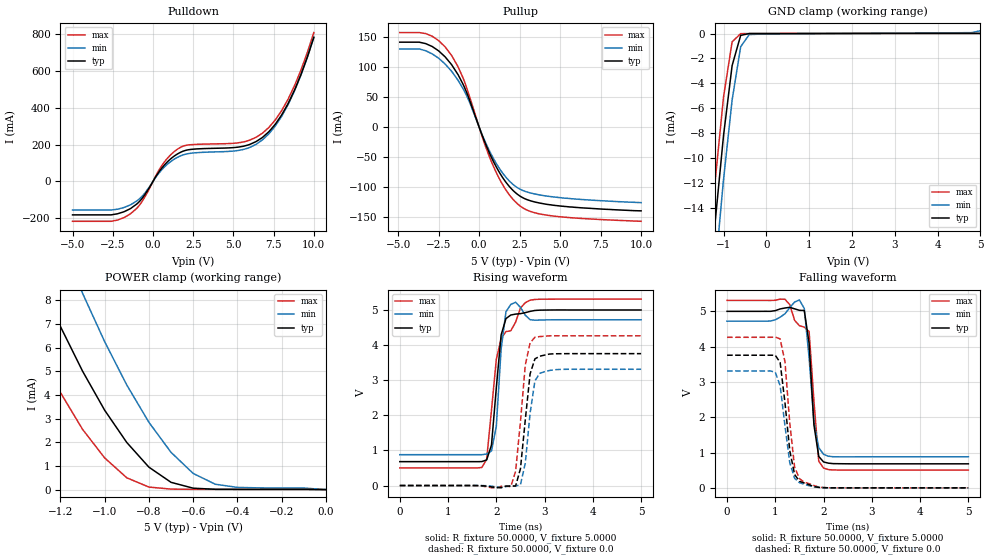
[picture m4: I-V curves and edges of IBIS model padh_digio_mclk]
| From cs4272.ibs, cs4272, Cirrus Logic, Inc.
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|   Model mclk
[Model]  padh_digio_mclk
Model_type I/O
Polarity   Non-Inverting
Enable   Active-High
Vinl =   0.8000V
Vinh =   2.0000V
C_comp   5.0000pF   5.0000pF   5.0000pF
[Temperature Range]   25.0000   85.0000   -40.0000
[Voltage Range]   5.0000V   4.5000V   5.5000V
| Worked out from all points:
|   slope of the pulldown table from 0 to 0.75 V, typ, clamps not added: 8.05 ohm
|   slope of the pullup table from 0 to 0.75 V, typ, clamps not added: 15.1 ohm
|   GND clamp passes 1 mA (typ) near -0.67 V on its own axis
|   POWER clamp passes 1 mA (typ) near -0.81 V on its own axis
|   rising waveform, R_fixture 50.0000, V_fixture 5.0000: 20-80 % time 166ps typ, 112ps min, 330ps max; typ from 0.681 V to 5 V
|   rising waveform, R_fixture 50.0000, V_fixture 0.0: 20-80 % time 167ps typ, 162ps min, 167ps max; typ from 0 V to 3.76 V
|   falling waveform, R_fixture 50.0000, V_fixture 5.0000: 20-80 % time 131ps typ, 149ps min, 154ps max; typ from 5 V to 0.681 V
|   falling waveform, R_fixture 50.0000, V_fixture 0.0: 20-80 % time 197ps typ, 189ps min, 169ps max; typ from 3.76 V to 0 V
[Pulldown]
|Voltage   I(typ)   I(min)   I(max)
-5V       -181.9mA   -155.7mA   -216.8mA
-2.6V     -181.9mA   -155.7mA   -216.8mA
-1.4V     -147.9mA   -127.4mA   -176.3mA
-700mV    -95.11mA   -83.14mA   -111.9mA
700mV     88.32mA    77.67mA    104.5mA
1.8V      162.1mA    142.1mA    189.6mA
5.5V      189.7mA    171.8mA    213.1mA
6.8V      239mA      225.7mA    262.3mA
7.6V      310.8mA    301.3mA    334.2mA
8.4V      423.9mA    418.1mA    447.7mA
9.2V      581.8mA    579.1mA    606.4mA
10V       784.4mA    784mA      810.2mA
[Pullup]
|Voltage   I(typ)   I(min)   I(max)
-4.9V     141.6mA    130.3mA    157.6mA
-3.7V     141.6mA    130.3mA    157.6mA
-2.9V     134.4mA    122.1mA    151.5mA
-1.7V     104.1mA    93.1mA     119.4mA
-900mV    65.98mA    59.32mA    75.33mA
300mV     -21.63mA   -19.83mA   -24.78mA
900mV     -58.13mA   -53.14mA   -66.4mA
1.7V      -93.45mA   -84.92mA   -106.6mA
2.5V      -114.5mA   -103mA     -130.8mA
3.2V      -123mA     -109.9mA   -140.8mA
4.5V      -129.8mA   -116mA     -147.9mA
10V       -139.5mA   -125.8mA   -156.9mA
[GND_clamp]
|Voltage   I(typ)   I(min)   I(max)
-5V       -173.1mA   -172.4mA   -178.6mA
-1.4V     -23.3mA    -27.39mA   -20.11mA
-1.2V     -15.29mA   -19.22mA   -11.99mA
-1V       -8.181mA   -11.72mA   -5.091mA
-800mV    -2.579mA   -5.348mA   -668.7uA
-600mV    -149.1uA   -1.06mA    -7.709uA
-400mV    -2.632uA   -83.68uA   -2.341uA
4.8V      8.423uA    72.58uA    11.35uA
5V        8.425uA    226.4uA    11.35uA
[POWER_clamp]
|Voltage   I(typ)   I(min)   I(max)
-5V       117.7mA    125.2mA    114.4mA
-1.4V     11.24mA    15.45mA    7.983mA
-1.3V     8.979mA    12.92mA    5.93mA
-1.2V     6.892mA    10.53mA    4.104mA
-1.1V     5.006mA    8.297mA    2.547mA
-1V       3.353mA    6.25mA     1.337mA
-900mV    1.99mA     4.419mA    498.5uA
-800mV    947.7uA    2.843mA    107.1uA
-700mV    307.4uA    1.574mA    20.85uA
-600mV    60.22uA    683.7uA    11.92uA
-400mV    8.755uA    94.23uA    11.37uA
0V        0A         0A         0A
[Ramp]
| variable   typ   min   max
dV/dt_r  2.2536/0.1653n   1.9014/0.2061n   2.6238/0.1453n
dV/dt_f  2.5910/0.1148n   2.2349/0.1350n   2.9499/95.1695p
R_load = 50.0000
[Rising Waveform]
R_fixture= 50.0000
V_fixture= 5.0000
V_fixture_min= 5.5000
V_fixture_max= 4.5000
|time   V(typ)   V(min)   V(max)
0s        680.7mV    879.7mV    503mV
1.7ns     682.4mV    879.6mV    514.6mV
1.8ns     729.8mV    895.7mV    749.8mV
1.9ns     1.152V     984.2mV    2.147V
2ns       2.78V      1.687V     3.591V
2.1ns     4.289V     3.884V     4.19V
2.2ns     4.753V     4.947V     4.383V
2.3ns     4.856V     5.157V     4.407V
2.7ns     4.959V     4.723V     5.278V
5ns       4.999V     4.72V      5.308V
[Rising Waveform]
R_fixture= 50.0000
V_fixture= 0.0
|time   V(typ)   V(min)   V(max)
0s        0V         315.2uV    0V
2.3ns     -17.24mV   -5.846mV   -27.79mV
2.4ns     -12.65mV   -11.01mV   404.1mV
2.5ns     478.1mV    23.41mV    1.815V
2.6ns     1.863V     633.4mV    3.425V
2.7ns     3.182V     2.06V      4.064V
2.8ns     3.607V     2.979V     4.221V
2.9ns     3.683V     3.194V     4.242V
3.3ns     3.753V     3.305V     4.264V
5ns       3.756V     3.311V     4.264V
[Falling Waveform]
R_fixture= 50.0000
V_fixture= 5.0000
V_fixture_min= 5.5000
V_fixture_max= 4.5000
|time   V(typ)   V(min)   V(max)
0s        4.999V     4.72V      5.308V
900ps     4.999V     4.724V     5.307V
1.2ns     5.093V     4.929V     5.34V
1.5ns     5.027V     5.321V     4.593V
1.6ns     5.023V     5.077V     4.55V
1.7ns     4.097V     3.689V     4.428V
1.8ns     1.783V     1.865V     2.466V
1.9ns     888.7mV    1.14V      754.3mV
2ns       734mV      948.4mV    560.4mV
5ns       680.7mV    879.3mV    503mV
[Falling Waveform]
R_fixture= 50.0000
V_fixture= 0.0
|time   V(typ)   V(min)   V(max)
0s        3.756V     3.311V     4.264V
900ps     3.756V     3.312V     4.264V
1ns       3.753V     3.273V     4.268V
1.1ns     3.549V     2.893V     4.219V
1.2ns     2.413V     1.76V      3.567V
1.3ns     1.05V      707.8mV    1.825V
1.4ns     378.5mV    269.4mV    583.2mV
1.6ns     138.8mV    101.9mV    161.3mV
2.1ns     2.124mV    992.9uV    2.022mV
5ns       2.712uV    0V         559.2nV
